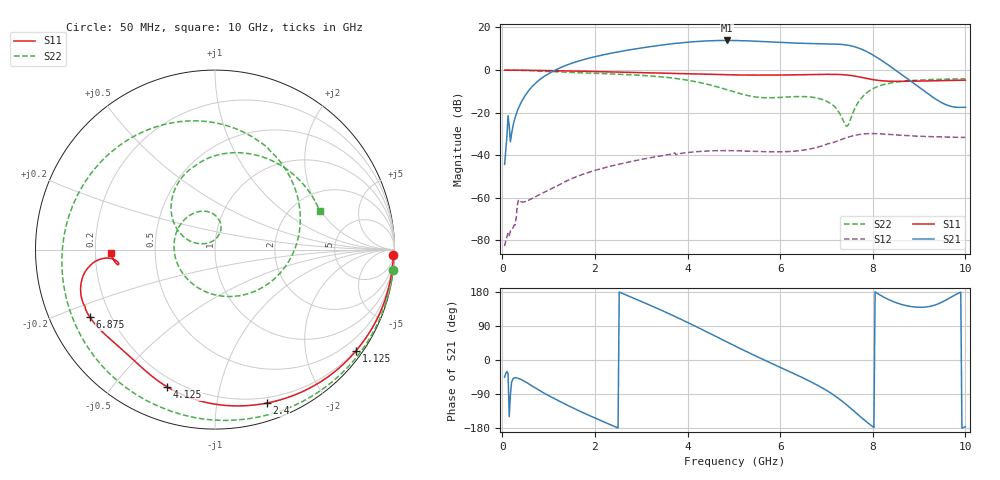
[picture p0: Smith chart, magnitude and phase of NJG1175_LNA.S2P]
! Created Fri Jun 18 20:03:53 2021
# hz S ma R 50
! 2 Port Network Data from SP1.SP block
! freq  magS11  angS11  magS21  angS21  magS12  angS12  magS22  angS22
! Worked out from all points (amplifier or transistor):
!   399 points, 50 MHz to 10 GHz, reference 50 ohm
!   highest |S21| = 13.9 dB at 4.85 GHz (marker M1)
!   |S21| within 3 dB of that: 3.165 GHz to 7.614 GHz (4.449 GHz wide, 82.5 % of centre)
!   unconditionally stable (mu >= 1): start of sweep to end of sweep
!   at 1.7 GHz: K = 2.98, MAG = 19.3 dB, |S12| = -49.3 dB
!   at 5.025 GHz: K = 3.15, MAG = 18.0 dB, |S12| = -37.9 dB
!   at 10 GHz: K = 57.84, MAG = -13.5 dB, |S12| = -31.7 dB
!   lowest NFmin = 0.49 dB at 1.275 GHz
!   S11 on the Smith chart (normalised r, x): 50 MHz: 14, -64; 1.125 GHz: 0.18, -3.09; 2.4 GHz: 0.15, -1.38; 4.125 GHz: 0.16, -0.70; 6.875 GHz: 0.12, -0.25; 10 GHz: 0.27, -0.02
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5e7  0.9935 -1.7  0.00608 -45.3  7.289e-05 -9.8  0.9997 -6.6
1.25e8  0.9944 -4.2  0.08518 -36.2  0.0001497 -61.5  0.9969 -16.5
1.75e8  0.9928 -5.7  0.02059 -91.5  0.0001649 -54.7  0.9959 -22.7
3.5e8  0.9911 -11.4  0.1277 -48.6  0.0008926 -70.5  0.9864 -44.8
1.125e9  0.9671 -35.8  0.9743 -102.0  0.001786 -175.9  0.9126 -125.0
1.725e9  0.9389 -53.4  1.722 -137.9  0.003511 150.8  0.8621 -169.9
2.4e9  0.9024 -71.4  2.551 -174.1  0.005735 118.5  0.8096 147.7
3.375e9  0.8511 -94.2  3.779 134.6  0.009434 79.6  0.7004 87.3
4.125e9  0.8104 -109.1  4.626 91.8  0.01192 46.9  0.546 32.7
4.475e9  0.7919 -115.2  4.87 70.6  0.01262 30.5  0.4505 2.4
4.85e9  0.7751 -121.0  4.96 47.6  0.01282 12.5  0.3463 -35.1
5.025e9  0.7692 -123.6  4.942 37.0  0.01274 4.2  0.3034 -55.1
5.775e9  0.7611 -133.8  4.591 -6.7  0.01201 -31.5  0.2231 -153.3
6.7e9  0.7864 -148.1  4.19 -59.8  0.01442 -86.9  0.2293 112.2
6.875e9  0.7925 -151.7  4.159 -71.3  0.01617 -100.9  0.2095 97.5
7.275e9  0.7873 -161.7  4.042 -102.9  0.02238 -139.5  0.1002 73.5
7.45e9  0.7629 -166.9  3.848 -119.8  0.0262 -159.1  0.04828 122.3
7.65e9  0.709 -172.2  3.412 -140.9  0.02988 176.5  0.1501 160.9
8e9  0.597 -175.5  2.272 -175.9  0.0322 136.1  0.3639 131.6
8.35e9  0.5464 -172.8  1.28 159.1  0.03074 105.3  0.4866 101.4
8.95e9  0.5504 -171.4  0.4324 139.4  0.02804 70.5  0.5779 64.3
1e10  0.5798 -177.9  0.1338 -176.2  0.02615 28.8  0.6218 20.0
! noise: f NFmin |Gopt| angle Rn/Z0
5e+07  2.437  0.9715  2.02  21.69
1.15e+09  0.4927  0.7616  29.9  0.3882
2.25e+09  0.5499  0.6661  52.92  0.2572
3.35e+09  0.6734  0.6107  75.21  0.2142
4.45e+09  0.8389  0.5775  96.41  0.1822
5.575e+09  1.05  0.5588  116.4  0.151
6.675e+09  1.283  0.5465  134.3  0.1197
7.775e+09  1.616  0.5389  151.5  0.09509
8.875e+09  4.795  0.626  162.9  0.1967
1e+10  12.18  0.6879  171.7  0.8555
